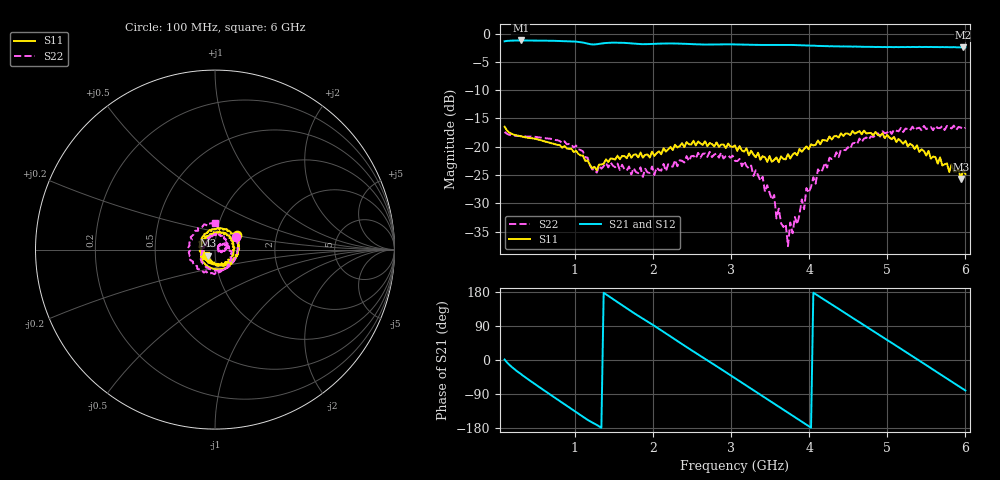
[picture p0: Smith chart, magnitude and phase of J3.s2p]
!Agilent Technologies,E8364B,MY43040379,A.07.50.67
!Agilent E8364B: A.07.50.67
!Date: Tuesday, March 24, 2026 10:38:14
!Correction: S11(Full 2 Port(1,2))
!S21(Full 2 Port(1,2))
!S12(Full 2 Port(1,2))
!S22(Full 2 Port(1,2))
!S2P File: Measurements: S11, S21, S12, S22:
# Hz S  dB  R 50
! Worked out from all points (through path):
!   201 points, 100 MHz to 6 GHz, reference 50 ohm
!   highest |S21| = -1.22 dB at 306.5 MHz (marker M1); lowest = -2.4 dB at 5.971 GHz (marker M2)
!   group delay of S21, straight-line fit = 371 ps
!   lowest |S11| = -25.7 dB at 5.941 GHz (marker M3), VSWR 1.11, Z = 46.1 - j3.12 ohm
!   |S11| at or under -10 dB: start of sweep to end of sweep
!   |S22| runs from -37.6 to -16.3 dB; largest |S21 - S12| = 0.0039
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1e8  -16.48 34.1  -1.37 1.2  -1.39 1.3  -17.40 31.2
3.065e8  -18.16 -27.5  -1.22 -36.9  -1.25 -36.9  -18.16 -27.2
6.9e8  -19.34 -93.2  -1.27 -92.1  -1.29 -92.1  -18.60 -89.5
1.103e9  -21.56 -160.8  -1.59 -150.1  -1.61 -150.1  -20.83 -155.4
1.28e9  -24.17 -172.0  -1.89 -171.3  -1.91 -171.3  -24.59 -161.8
1.5455e9  -21.59 159.6  -1.61 152.7  -1.62 152.7  -22.99 173.8
2.0765e9  -20.83 96.2  -1.78 82.2  -1.79 82.2  -24.15 134.1
2.5485e9  -19.78 38.5  -1.90 18.3  -1.93 18.3  -22.10 97.6
3.05e9  -19.79 -33.5  -1.91 -48.1  -1.92 -48.2  -22.51 31.9
3.5515e9  -22.33 -127.7  -2.01 -114.9  -2.02 -114.8  -28.56 -21.8
3.581e9  -21.90 -141.5  -2.01 -118.9  -2.02 -118.9  -32.69 -15.3
3.699e9  -22.23 -163.2  -2.01 -134.8  -2.02 -134.7  -33.67 -15.5
3.7285e9  -21.32 -174.7  -2.02 -138.8  -2.03 -138.8  -37.59 23.8
3.758e9  -22.10 177.2  -2.01 -142.8  -2.04 -142.8  -33.40 19.6
3.8465e9  -21.52 160.9  -2.04 -154.8  -2.07 -154.7  -33.75 31.3
4.053e9  -19.80 114.3  -2.14 177.6  -2.16 177.7  -25.43 32.9
4.584e9  -17.69 34.2  -2.30 107.5  -2.33 107.5  -19.31 -37.4
5.0265e9  -18.39 -24.2  -2.38 49.2  -2.41 49.2  -17.08 -107.4
5.469e9  -20.78 -77.3  -2.38 -9.5  -2.39 -9.5  -16.34 177.6
5.941e9  -25.69 -139.4  -2.43 -72.7  -2.45 -72.6  -16.62 96.0
5.9705e9  -24.10 -138.6  -2.45 -76.6  -2.46 -76.5  -16.91 95.1
6e9  -24.84 -147.8  -2.43 -80.5  -2.46 -80.4  -16.65 89.5
